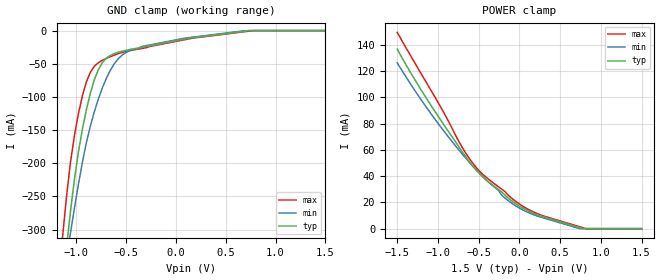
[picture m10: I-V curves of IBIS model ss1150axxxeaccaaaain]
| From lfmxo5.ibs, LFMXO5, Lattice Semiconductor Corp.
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|   Model   ss1150axxxeaccaaaain
[Model] ss1150axxxeaccaaaain
Model_type   Input
Polarity   Non-Inverting
Vinl   =   0.650V
Vinh   =   0.850V
C_comp  4.383pF 4.308pF 4.470pF
[Model Spec]
| Input threshold voltage corners
Vinl  0.5750V  0.5375V  0.6125V
Vinh  0.9250V  0.8875V  0.9625V
[Receiver Thresholds]
Vth  =  0.750V
Vth_min  =  0.735V
Vth_max  =  0.765V
Vinh_ac  =  0.175V
Vinh_dc  =  0.100V
Vinl_ac  = -0.175V
Vinl_dc  = -0.100V
Tslew_ac =  5.000ns |Not specified, so set to high value"
[Temperature Range]   25   0.125k  -40
[Voltage Range] 1.500V  1.430V  1.580V
[GND_clamp]
|Voltage   I(typ)  I(min)  I(max)
-1.5V     -999.5mA   -804.2mA   -1.074A
-1.14V    -384.5mA   -384.9mA   -312.4mA
-1.1V     -327.1mA   -344.3mA   -250.9mA
-1.06V    -273mA     -305.2mA   -198.7mA
-1.02V    -224mA     -267.7mA   -158.2mA
-940mV    -148.7mA   -198.5mA   -98.27mA
-860mV    -94.3mA    -143.9mA   -62.84mA
-780mV    -58.91mA   -103.3mA   -48.5mA
-580mV    -32.8mA    -42.44mA   -34.81mA
-340mV    -25.17mA   -23.9mA    -26.9mA
780mV     0A         0A         -74.81uA
1.5V      0A         0A         0A
[POWER_clamp]
|Voltage   I(typ)  I(min)  I(max)
-1.5V     136.8mA    126.4mA    149.6mA
-1.06V    91.57mA    85.46mA    102.8mA
-740mV    62.22mA    59.81mA    66.12mA
-620mV    51.61mA    51.02mA    54mA
-460mV    40.23mA    40.21mA    42.05mA
-260mV    29.96mA    29.4mA     32.05mA
-220mV    28.14mA    25.72mA    30.23mA
-60mV     19.65mA    17.96mA    21.49mA
260mV     9.583mA    8.846mA    10.48mA
740mV     737uA      0A         1.474mA
820mV     0A         0A         0A
1.5V      0A         0A         0A
